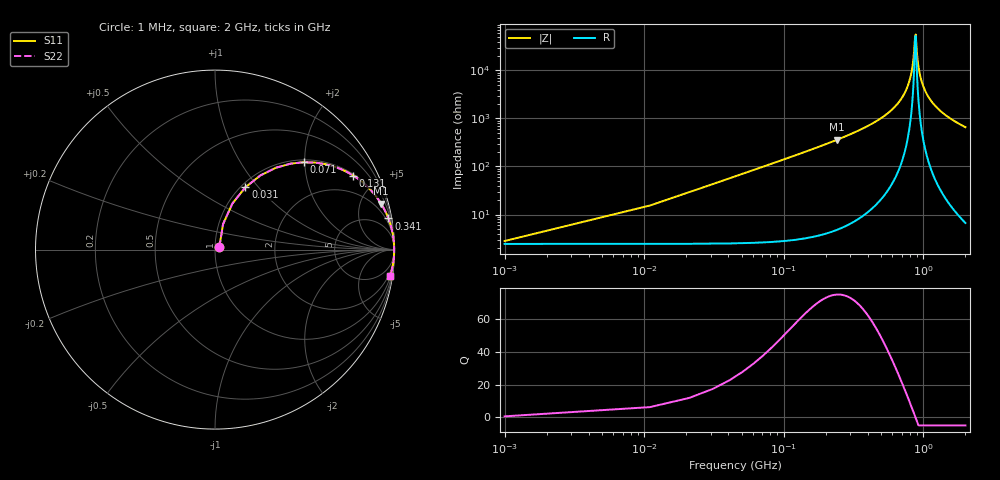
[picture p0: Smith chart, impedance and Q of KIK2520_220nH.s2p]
!version-2
!date-01.2022
!Series
# MHz S RI R 50
!Freq ReS11 ImS11 ReS21 ImS21 ReS12 ImS12 ReS22 ImS22
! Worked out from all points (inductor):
!   201 points, 1 MHz to 2 GHz, reference 50 ohm
!   read as one part in series: L = 220 nH near 11 MHz
!   highest Q = 74.9 at 241 MHz (marker M1), where L = 238 nH
!   self-resonance near 871 MHz
!   S11 on the Smith chart (normalised r, x): 1 MHz: 1.05, +0.03; 31 MHz: 1.05, +0.86; 71 MHz: 1.05, +1.98; 131 MHz: 1.06, +3.70; 341 MHz: 1, +11; 2 GHz: 1, -13
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1  0.024 0.0132  0.976 -0.0132  0.976 -0.0132  0.024 0.0132
11  0.0449 0.1418  0.9551 -0.1418  0.9551 -0.1418  0.0449 0.1418
21  0.0966 0.2561  0.9034 -0.2561  0.9034 -0.2561  0.0966 0.2561
31  0.1697 0.3476  0.8303 -0.3476  0.8303 -0.3476  0.1697 0.3476
71  0.4942 0.4869  0.5058 -0.4869  0.5058 -0.4869  0.4942 0.4869
131  0.7705 0.4123  0.2295 -0.4123  0.2295 -0.4123  0.7705 0.4123
241  0.9256 0.2559  0.0744 -0.2559  0.0744 -0.2559  0.9256 0.2559
341  0.9662 0.1736  0.0338 -0.1736  0.0338 -0.1736  0.9662 0.1736
671  0.9962 0.0445  0.00377 -0.0445  0.00377 -0.0445  0.9962 0.0445
751  0.9976 0.0257  0.00238 -0.0257  0.00238 -0.0257  0.9976 0.0257
811  0.9981 0.013  0.00186 -0.013  0.00186 -0.013  0.9981 0.013
841  0.9983 0.007  0.00173 -0.007  0.00173 -0.007  0.9983 0.007
871  0.9983 0.00124  0.00167 -0.00124  0.00167 -0.00124  0.9983 0.00124
881  0.9983 -0.000639  0.00166 0.000639  0.00166 0.000639  0.9983 -0.000639
901  0.9983 -0.00433  0.00167 0.00433  0.00167 0.00433  0.9983 -0.00433
921  0.9983 -0.00794  0.00171 0.00794  0.00171 0.00794  0.9983 -0.00794
951  0.9982 -0.0132  0.00181 0.0132  0.00181 0.0132  0.9982 -0.0132
1001  0.9979 -0.0217  0.00209 0.0217  0.00209 0.0217  0.9979 -0.0217
1131  0.9966 -0.0421  0.00337 0.0421  0.00337 0.0421  0.9966 -0.0421
1341  0.9933 -0.0714  0.0067 0.0714  0.0067 0.0714  0.9933 -0.0714
1671  0.9858 -0.1119  0.0142 0.1119  0.0142 0.1119  0.9858 -0.1119
2000  0.9761 -0.1478  0.0239 0.1478  0.0239 0.1478  0.9761 -0.1478
